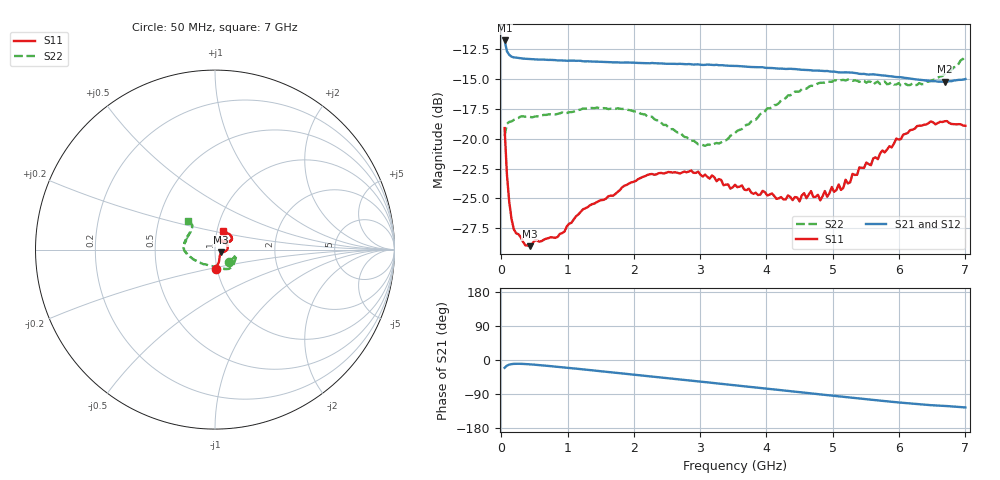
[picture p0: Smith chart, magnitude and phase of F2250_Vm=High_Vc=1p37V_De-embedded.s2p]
! Integrated Device Technology
! Corporate Headquarters
! 6024 Silver Creek Valley Road
! San Jose, CA 95138  USA
! Phone:  1-408-284-8200
! Toll Free:  1-800-223-1366
! Webpage:  http://www.idt.com/
! Timing and RF Division
! 515 Groton Road, Suite 102
! Westford, MA 01886-6024
! Device:  F2250
! Description: Voltage Variable RF Attenuator
! Frequency:  50.0 -  6000.00 MHz
! Package:  3x3 mm Thin QFN Plastic Package: 16 pin
! Ports:  2 RF, 3 DC
!  Pin  1  = GND
!  Pin  2  = NC
!  Pin  3  = RF1  = Port 1
!  Pin  4  = NC
!  Pin  5  = GND
!  Pin  6  = GND
!  Pin  7  = GND
!  Pin  8  = GND
!  Pin  9  = NC
!  Pin 10  = RF2  = Port 2
!  Pin 11  = NC
!  Pin 12  = GND
!  Pin 13  = GND
!  Pin 14  = VCNTRL
!  Pin 15  = VDD
!  Pin 16  = VMODE
! Vcntrl:  1.370 Volts
! Vmode:  +3.300 Volts
! Vdd:  +3.30  Volts
! Current:  1.333 mA
! Data:  The device was measured on a the F2250 evaluation board which has
!  individual transmission lines to the RF pins.  Data was collected
!  using a calibrated network analyzer.  The evaluation board was
!  de-embedded using a TRL calibration technique.
!  The reference plane is the edge of the package pin.
! Misc:  SN 10
!  Action Tracker AT0258
! Date Measured:  2014-11-26
! Date:  2015-10-15  MJV
! Note:
!  Integrated Device Technology supplies this data as a sample of measured
!  data at the package pin for this product.  Your particular data for this
!  product may vary.
!  Data was taken at 25 degrees C.
!  Integrated Device Technology reserves the right to change this data at anytime.
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# GHz S dB R 50
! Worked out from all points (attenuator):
!   201 points, 50 MHz to 7 GHz, reference 50 ohm
!   highest |S21| = -11.77 dB at 50 MHz (marker M1); lowest = -15.2 dB at 6.687 GHz (marker M2)
!   lowest |S11| = -29.0 dB at 432.2 MHz (marker M3), VSWR 1.07, Z = 53.3 - j1.64 ohm
!   |S11| at or under -10 dB: start of sweep to end of sweep
!   |S22| runs from -20.6 to -13.1 dB; largest |S21 - S12| = 0.00084
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0.05  -19.11 -88.0  -11.77 -20.5  -11.77 -20.5  -19.77 -40.4
0.08475  -22.98 -71.8  -12.68 -14.9  -12.67 -14.8  -18.75 -21.5
0.15425  -26.73 -55.8  -13.13 -10.9  -13.11 -10.8  -18.55 -14.3
0.22375  -27.93 -41.7  -13.21 -10.0  -13.21 -10.0  -18.34 -14.3
0.43225  -29.00 -25.7  -13.34 -11.4  -13.35 -11.4  -18.17 -16.6
0.84925  -28.23 -17.6  -13.45 -18.0  -13.44 -18.0  -17.92 -30.2
1.2315  -25.92 -15.4  -13.52 -24.7  -13.52 -24.7  -17.48 -40.2
2.37825  -22.88 7.6  -13.69 -45.3  -13.68 -45.4  -18.45 -65.2
3.07325  -23.01 28.6  -13.82 -58.3  -13.82 -58.3  -20.60 -100.7
3.525  -23.86 44.7  -13.91 -66.8  -13.92 -66.8  -19.53 -131.9
4.1505  -25.04 62.8  -14.12 -78.4  -14.11 -78.4  -17.17 -160.9
4.7065  -24.89 60.8  -14.30 -88.8  -14.27 -88.8  -15.58 -175.7
4.81075  -25.16 56.6  -14.31 -90.7  -14.30 -90.7  -15.32 -177.7
5.08875  -23.83 47.7  -14.44 -95.8  -14.42 -95.9  -15.17 175.9
5.1235  -24.29 47.8  -14.45 -96.5  -14.43 -96.6  -15.10 174.9
5.193  -23.44 42.8  -14.44 -97.8  -14.44 -97.8  -15.12 173.7
5.2625  -23.65 38.6  -14.47 -99.1  -14.46 -99.1  -15.05 172.7
5.4015  -22.40 36.2  -14.57 -101.6  -14.55 -101.7  -15.24 168.4
5.85325  -20.63 29.7  -14.77 -109.6  -14.77 -109.7  -15.40 156.8
6.27025  -18.95 32.3  -15.04 -116.4  -15.03 -116.5  -15.50 143.6
6.68725  -18.54 45.0  -15.23 -121.3  -15.25 -121.3  -14.57 132.8
7  -18.92 65.8  -15.00 -125.2  -15.03 -125.3  -13.11 133.3
